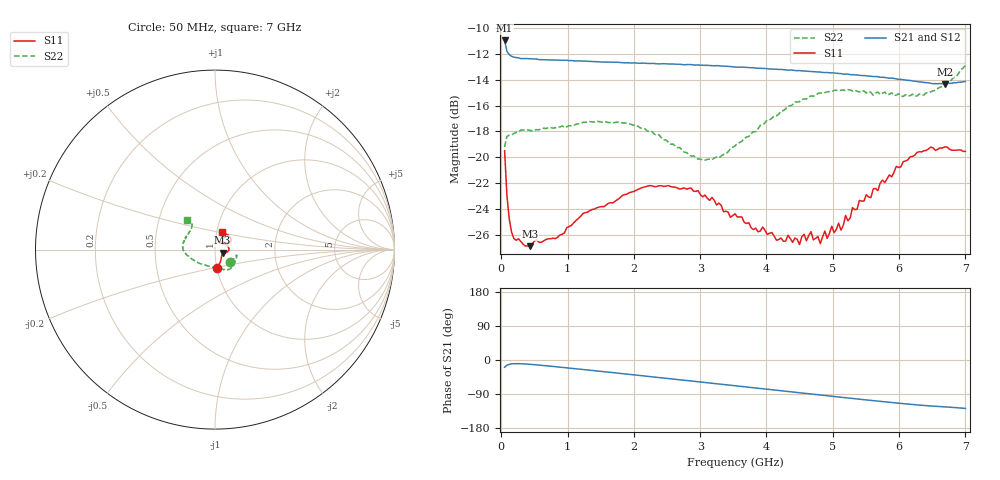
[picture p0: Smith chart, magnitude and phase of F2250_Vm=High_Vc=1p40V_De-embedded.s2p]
! Integrated Device Technology
! Corporate Headquarters
! 6024 Silver Creek Valley Road
! San Jose, CA 95138  USA
! Phone:  1-408-284-8200
! Toll Free:  1-800-223-1366
! Webpage:  http://www.idt.com/
! Timing and RF Division
! 515 Groton Road, Suite 102
! Westford, MA 01886-6024
! Device:  F2250
! Description: Voltage Variable RF Attenuator
! Frequency:  50.0 -  6000.00 MHz
! Package:  3x3 mm Thin QFN Plastic Package: 16 pin
! Ports:  2 RF, 3 DC
!  Pin  1  = GND
!  Pin  2  = NC
!  Pin  3  = RF1  = Port 1
!  Pin  4  = NC
!  Pin  5  = GND
!  Pin  6  = GND
!  Pin  7  = GND
!  Pin  8  = GND
!  Pin  9  = NC
!  Pin 10  = RF2  = Port 2
!  Pin 11  = NC
!  Pin 12  = GND
!  Pin 13  = GND
!  Pin 14  = VCNTRL
!  Pin 15  = VDD
!  Pin 16  = VMODE
! Vcntrl:  1.400 Volts
! Vmode:  +3.300 Volts
! Vdd:  +3.30  Volts
! Current:  1.331 mA
! Data:  The device was measured on a the F2250 evaluation board which has
!  individual transmission lines to the RF pins.  Data was collected
!  using a calibrated network analyzer.  The evaluation board was
!  de-embedded using a TRL calibration technique.
!  The reference plane is the edge of the package pin.
! Misc:  SN 10
!  Action Tracker AT0258
! Date Measured:  2014-11-26
! Date:  2015-10-15  MJV
! Note:
!  Integrated Device Technology supplies this data as a sample of measured
!  data at the package pin for this product.  Your particular data for this
!  product may vary.
!  Data was taken at 25 degrees C.
!  Integrated Device Technology reserves the right to change this data at anytime.
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# GHz S dB R 50
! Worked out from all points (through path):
!   201 points, 50 MHz to 7 GHz, reference 50 ohm
!   highest |S21| = -10.96 dB at 50 MHz (marker M1); lowest = -14.3 dB at 6.687 GHz (marker M2)
!   group delay of S21, straight-line fit = 50.6 ps
!   lowest |S11| = -26.9 dB at 432.2 MHz (marker M3), VSWR 1.09, Z = 54.4 - j1.78 ohm
!   |S11| at or under -10 dB: start of sweep to end of sweep
!   |S22| runs from -20.2 to -12.9 dB; largest |S21 - S12| = 0.00099
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0.05  -19.50 -83.1  -10.96 -19.0  -10.97 -19.0  -19.20 -40.1
0.08475  -22.94 -63.6  -11.80 -13.7  -11.79 -13.7  -18.38 -21.9
0.15425  -25.78 -45.2  -12.18 -10.2  -12.18 -10.2  -18.26 -14.8
0.43225  -26.88 -21.2  -12.38 -11.3  -12.39 -11.3  -17.92 -17.1
0.84925  -26.19 -17.4  -12.48 -18.2  -12.48 -18.2  -17.70 -30.9
1.2315  -24.35 -17.0  -12.55 -25.1  -12.58 -25.1  -17.29 -41.1
2.37825  -22.20 1.9  -12.77 -46.1  -12.77 -46.2  -18.26 -67.0
3.0385  -23.05 19.6  -12.87 -58.7  -12.90 -58.7  -20.22 -100.1
3.525  -24.37 36.6  -13.02 -68.0  -13.01 -68.0  -19.12 -133.4
4.1505  -26.41 56.6  -13.19 -79.9  -13.19 -79.9  -16.79 -161.9
4.498  -26.75 55.3  -13.29 -86.5  -13.28 -86.5  -15.70 -172.4
4.67175  -25.76 56.0  -13.36 -89.8  -13.38 -89.8  -15.25 -176.2
4.7065  -26.38 56.5  -13.38 -90.4  -13.39 -90.4  -15.28 -176.8
4.81075  -26.68 51.8  -13.40 -92.4  -13.43 -92.3  -15.02 -178.7
4.88025  -25.71 49.5  -13.44 -93.7  -13.45 -93.7  -15.00 179.2
5.08875  -25.09 43.0  -13.51 -97.6  -13.51 -97.7  -14.87 174.7
5.1235  -25.63 42.9  -13.53 -98.3  -13.54 -98.3  -14.81 173.7
5.29725  -23.89 34.0  -13.62 -101.4  -13.60 -101.5  -14.87 170.3
5.85325  -21.37 26.5  -13.88 -111.5  -13.87 -111.7  -15.13 155.3
6.27025  -19.62 30.4  -14.13 -118.5  -14.14 -118.5  -15.25 142.2
6.68725  -19.19 44.8  -14.32 -123.6  -14.32 -123.8  -14.36 131.9
7  -19.54 67.6  -14.13 -127.8  -14.13 -127.9  -12.89 132.6
